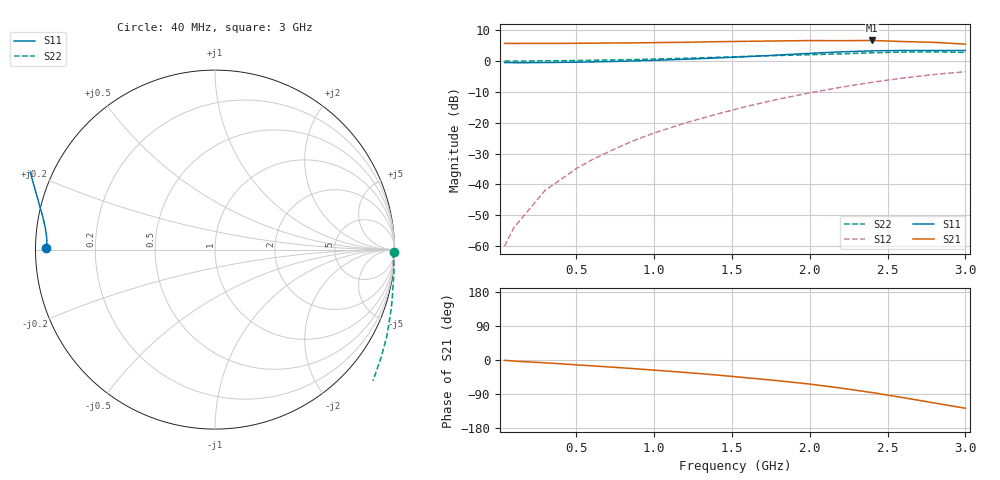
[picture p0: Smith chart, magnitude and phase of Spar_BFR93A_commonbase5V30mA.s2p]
! Filename:  BFR93ACD.S2P  Version:  2.0
! NXP part #: BFR93A  Date: Jul 1990
! Bias condition: Vce=5V, Ic=30mA
! COMMON BASE
#  MHz  S  MA  R  50
! Freq  S11  S21  S12  S22
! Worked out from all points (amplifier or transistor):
!   21 points, 40 MHz to 3 GHz, reference 50 ohm
!   highest |S21| = 6.6 dB at 2.4 GHz (marker M1)
!   |S21| within 3 dB of that: start of sweep to end of sweep
!   unconditionally stable (mu >= 1): nowhere
!   at 300 MHz: K = -0.68, MSG = 23.8 dB, |S12| = -41.9 dB
!   at 1 GHz: K = -0.94, MSG = 14.6 dB, |S12| = -23.3 dB
!   at 3 GHz: K = -0.86, MSG = 4.5 dB, |S12| = -3.5 dB
40  0.94 179.3  1.922 -0.9  0.001 49.6  0.995 -0.9
100  0.938 178.2  1.92 -2.8  0.002 80.6  0.994 -2.7
200  0.938 176.8  1.924 -5.2  0.004 109.2  0.999 -5.0
300  0.942 175.3  1.923 -7.5  0.008 128.3  1.006 -7.5
400  0.948 173.9  1.923 -10.0  0.012 133.9  1.009 -10.2
500  0.954 172.5  1.933 -12.8  0.018 138.9  1.016 -12.9
600  0.964 171.0  1.94 -15.4  0.025 142.0  1.025 -15.6
700  0.976 169.3  1.95 -18.1  0.033 143.7  1.035 -18.4
800  0.99 167.7  1.955 -20.8  0.043 144.8  1.045 -21.2
900  1.006 166.1  1.965 -23.7  0.055 145.3  1.057 -23.9
1000  1.023 164.4  1.98 -26.8  0.068 144.8  1.073 -26.9
1200  1.065 160.9  2.006 -32.8  0.099 143.5  1.104 -33.1
1400  1.117 157.2  2.05 -39.5  0.137 140.7  1.144 -39.7
1600  1.175 152.8  2.078 -47.1  0.185 137.9  1.186 -46.8
1800  1.248 147.8  2.11 -54.8  0.241 133.1  1.224 -54.8
2000  1.327 142.4  2.137 -63.6  0.304 127.7  1.263 -63.8
2200  1.403 136.7  2.128 -74.1  0.375 121.5  1.301 -74.6
2400  1.456 129.7  2.147 -85.9  0.451 113.7  1.356 -86.1
2600  1.481 121.6  2.062 -99.3  0.529 105.4  1.394 -97.7
2800  1.478 112.0  1.999 -113.4  0.603 96.2  1.406 -109.4
3000  1.475 102.4  1.87 -127.3  0.669 88.3  1.372 -121.0
